(* Logix 5000 AddOnInstructionDefinition export ACS_HOME_HERE; software revision 24.00 *)

ADD_ON_INSTRUCTION ACS_HOME_HERE   (* revision 1.1, vendor Tolomatic, Inc. *)
// Enable and Declare Current Position Home
// Revision note:
// Previous version used a timer and the home command to simulate this function.  Firmware now supports a Home Here Command (0x15) in the command register to support this directly.
VAR_IN_OUT
   DriveCMD : SINT; {required}   // ACS.O.CMD
END_VAR

ROUTINE Logic   (* ladder *)
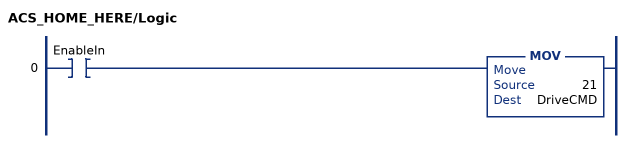
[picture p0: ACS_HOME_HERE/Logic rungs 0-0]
   0: XIC(EnableIn)MOV(21,DriveCMD);
END_ROUTINE
END_ADD_ON_INSTRUCTION
